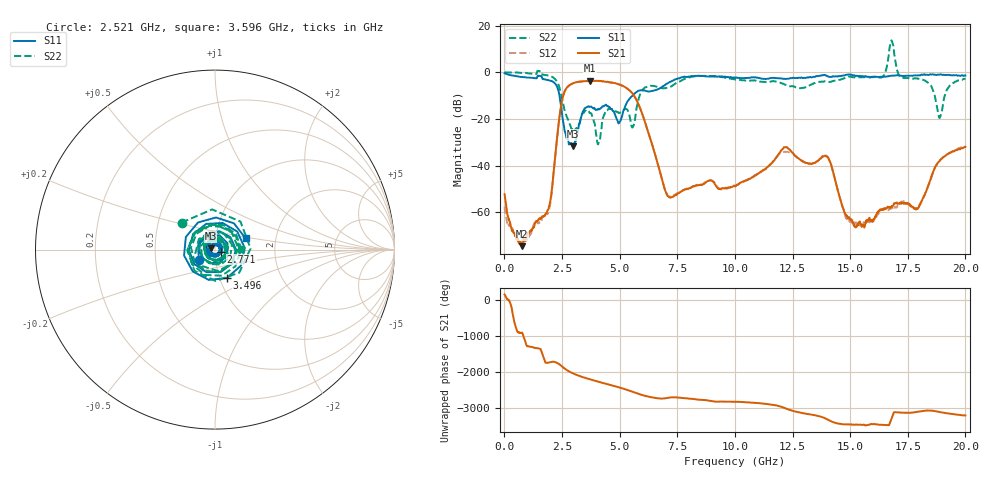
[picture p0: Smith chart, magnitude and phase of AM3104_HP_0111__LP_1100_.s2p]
!Created with skrf (http://scikit-rf.org).
# Hz S RI R 50.0
!freq ReS11 ImS11 ReS21 ImS21 ReS12 ImS12 ReS22 ImS22
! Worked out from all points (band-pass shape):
!   1601 points, 10 MHz to 20 GHz, reference 50 ohm
!   highest |S21| = -3.65 dB at 3.708 GHz (marker M1); lowest = -74.4 dB at 759.6 MHz (marker M2)
!   |S21| within 3 dB of the highest: 2.706 GHz to 5.285 GHz (2.579 GHz wide, 64.6 % of centre)
!   lowest |S11| = -31.7 dB at 2.984 GHz (marker M3), VSWR 1.05, Z = 47.6 + j0.742 ohm
!   |S11| at or under -10 dB: 2.391 GHz to 5.561 GHz (3.171 GHz wide, 79.7 % of centre)
!   |S22| runs from -30.8 to 13.6 dB; largest |S21 - S12| = 0.057
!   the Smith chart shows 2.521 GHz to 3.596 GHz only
!   S11 on the Smith chart (normalised r, x): 2.521 GHz: 0.83, -0.10; 2.771 GHz: 1.07, -0.02; 3.496 GHz: 1.08, -0.35; 3.596 GHz: 1.40, +0.18
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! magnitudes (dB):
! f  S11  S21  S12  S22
! 10 MHz  -0.4  -52.2  -57.5  0.0
! 759.6 MHz  -2.0  -74.4  -72.4  -0.3
! 1.922 GHz  -3.4  -58.1  -59.3  -1.4
! 2.521 GHz  -19.4  -11.2  -11.2  -12.4
! 2.771 GHz  -29.2  -6.0  -6.0  -20.5
! 2.984 GHz  -31.7  -4.6  -4.7  -24.8
! 3.346 GHz  -18.7  -3.9  -4.0  -18.9
! 3.496 GHz  -15.3  -3.8  -3.8  -16.5
! 3.596 GHz  -14.8  -3.7  -3.8  -16.7
! 3.708 GHz  -14.8  -3.6  -3.7  -17.4
! 4.07 GHz  -15.7  -3.7  -3.7  -30.8
! 5.545 GHz  -10.2  -8.9  -8.9  -23.6
! 6.682 GHz  -7.2  -40.1  -40.2  -6.3
! 7.181 GHz  -4.1  -53.6  -53.2  -6.3
! 10.01 GHz  -2.4  -48.8  -48.8  -3.1
! 13.34 GHz  -2.1  -39.2  -39.2  -5.1
! 14.04 GHz  -1.8  -36.5  -36.5  -4.1
! 15.21 GHz  -1.5  -66.2  -64.4  -2.2
! 16.68 GHz  -1.6  -57.7  -58.9  7.3
! 17.93 GHz  -1.3  -58.5  -57.8  -2.7
! 18.89 GHz  -1.0  -37.8  -37.9  -19.5
! 20 GHz  -1.4  -32.0  -31.4  -2.7
